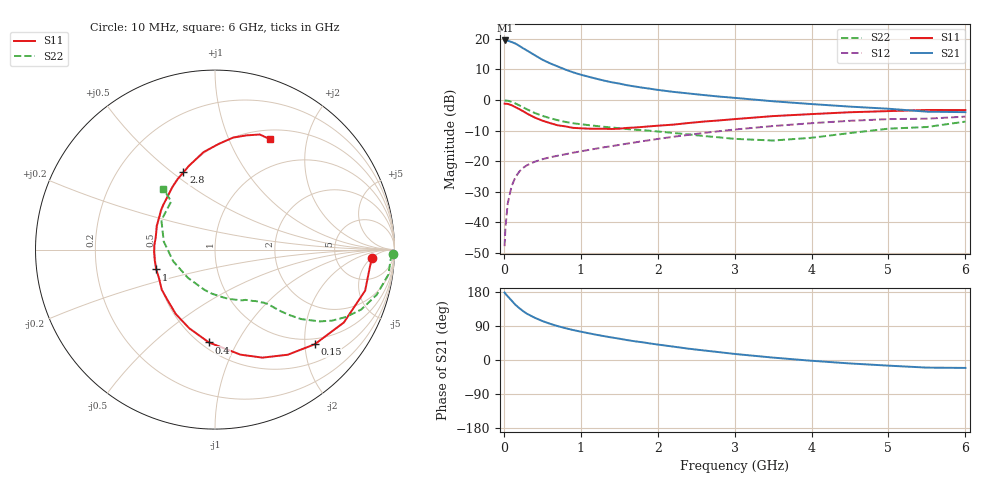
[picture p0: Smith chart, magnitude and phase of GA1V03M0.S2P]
! Infineon Technologies  Discrete & RF Semiconductors
! BF775
! Si NPN RF Bipolar Junction Transistor in SOT23
! VCE = 1 V  IC = 3 mA
! Common Emitter S-Parameters:  May  1996
# GHz  S  MA  R  50
!  f  S11  S21  S12  S22
! GHz  MAG  ANG  MAG  ANG  MAG  ANG  MAG  ANG
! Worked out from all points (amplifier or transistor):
!   36 points, 10 MHz to 6 GHz, reference 50 ohm
!   highest |S21| = 19.5 dB at 20 MHz (marker M1)
!   |S21| within 3 dB of that: start of sweep to 281.1 MHz
!   unconditionally stable (mu >= 1): 895.3 MHz to end of sweep
!   at 250 MHz: K = 0.38, MSG = 19.5 dB, |S12| = -22.2 dB
!   at 1.4 GHz: K = 1.18, MAG = 7.9 dB, |S12| = -15.1 dB
!   at 6 GHz: K = 1.04, MAG = -0.5 dB, |S12| = -5.4 dB
!   S11 on the Smith chart (normalised r, x): 10 MHz: 13, -5; 150 MHz: 0.87, -2.22; 400 MHz: 0.55, -0.77; 1 GHz: 0.50, -0.12; 2.8 GHz: 0.50, +0.55; 6 GHz: 0.61, +1.43
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0.01  0.8761 -3.0  9.306 177.9  0.0041 87.7  0.9928 -1.5
0.02  0.8686 -6.2  9.41 175.0  0.0079 89.2  0.9802 -3.2
0.05  0.8672 -15.3  9.357 168.1  0.0202 81.5  0.9759 -8.2
0.1  0.8248 -29.5  8.876 157.1  0.0389 73.9  0.9355 -15.6
0.15  0.766 -43.5  8.384 145.7  0.0548 66.7  0.8803 -22.3
0.2  0.7124 -55.3  7.694 137.1  0.0676 61.3  0.8198 -27.3
0.25  0.6573 -66.3  7.016 129.1  0.0779 56.7  0.762 -31.3
0.3  0.6021 -76.4  6.456 122.1  0.086 53.5  0.7063 -34.5
0.4  0.5186 -93.7  5.42 111.7  0.0981 48.9  0.6163 -38.9
0.5  0.4613 -108.1  4.568 102.9  0.1078 46.4  0.5529 -41.3
0.6  0.4207 -121.2  3.988 95.7  0.1161 45.0  0.5057 -43.0
0.7  0.3868 -132.9  3.539 89.4  0.1231 44.7  0.4688 -44.2
0.8  0.3712 -143.2  3.147 84.0  0.1302 44.6  0.4396 -45.2
1  0.3458 -161.4  2.596 74.8  0.1452 44.7  0.4029 -47.3
1.1  0.341 -169.5  2.407 70.7  0.1531 44.8  0.3895 -48.9
1.6  0.3506 157.8  1.749 52.6  0.1938 45.3  0.3364 -56.9
2.2  0.3965 131.8  1.362 35.4  0.2507 43.1  0.2904 -71.9
2.8  0.4648 112.2  1.14 20.7  0.3098 38.1  0.2458 -94.3
3.5  0.5469 96.7  0.955 6.3  0.3762 30.2  0.2181 -133.6
4.5  0.6322 80.8  0.781 -9.1  0.4581 17.3  0.2891 171.0
5.5  0.6883 68.7  0.646 -20.1  0.4961 3.2  0.3627 132.3
6  0.6865 63.7  0.634 -20.9  0.5358 -0.7  0.4446 130.3
